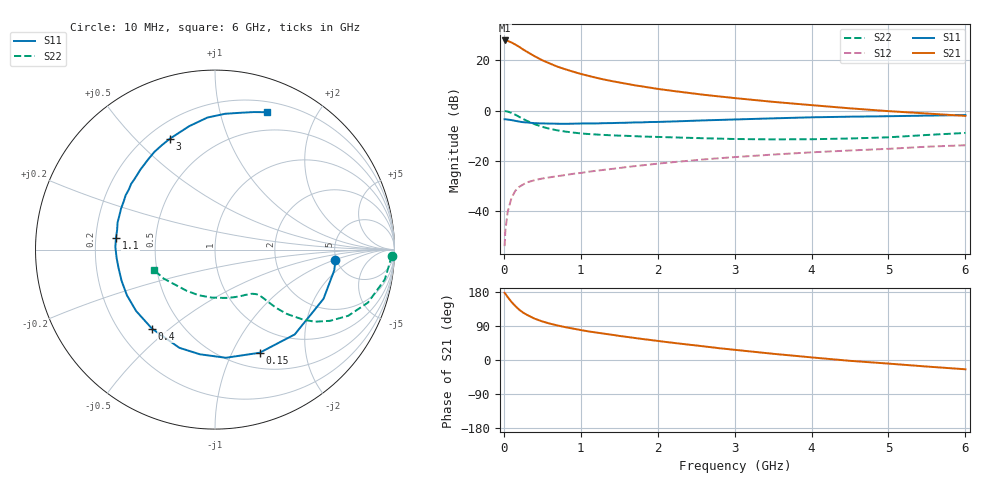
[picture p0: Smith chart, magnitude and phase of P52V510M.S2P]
! SIEMENS Small Signal Semiconductors
! BFP183
! Si NPN RF Bipolar Junction Transistor in SOT143
! VCE = 2.5 V  IC = 10 mA
! Common Emitter S-Parameters:  March  1996
# GHz  S  MA  R  50
!  f  S11  S21  S12  S22
! GHz  MAG  ANG  MAG  ANG  MAG  ANG  MAG  ANG
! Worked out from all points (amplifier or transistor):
!   36 points, 10 MHz to 6 GHz, reference 50 ohm
!   highest |S21| = 28.0 dB at 10 MHz (marker M1)
!   |S21| within 3 dB of that: start of sweep to 222.3 MHz
!   unconditionally stable (mu >= 1): 1.144 GHz to 5.571 GHz
!   at 250 MHz: K = 0.33, MSG = 26.9 dB, |S12| = -29.4 dB
!   at 1.4 GHz: K = 1.09, MAG = 15.7 dB, |S12| = -23.2 dB
!   at 6 GHz: K = 0.95, MSG = 5.8 dB, |S12| = -13.8 dB
!   lowest NFmin = 1.30 dB at 450 MHz
!   S11 on the Smith chart (normalised r, x): 10 MHz: 4.91, -1.01; 150 MHz: 0.68, -1.28; 400 MHz: 0.34, -0.44; 1.1 GHz: 0.29, +0.05; 3 GHz: 0.29, +0.63; 6 GHz: 0.30, +1.40
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0.01  0.6737 -4.8  25.01 177.2  0.002 82.8  0.9842 -2.0
0.02  0.6744 -9.8  24.98 174.7  0.0041 85.6  0.9774 -4.1
0.05  0.6639 -24.4  24.54 166.0  0.0097 79.9  0.9605 -10.0
0.1  0.6486 -46.8  22.76 153.2  0.0184 68.8  0.9021 -19.1
0.15  0.6262 -66.6  20.7 142.1  0.0254 60.9  0.829 -26.4
0.2  0.6057 -84.3  18.67 132.7  0.0303 55.9  0.7533 -31.8
0.25  0.5893 -98.2  16.57 125.1  0.0338 51.0  0.685 -35.9
0.3  0.5821 -109.9  14.9 119.3  0.0373 47.8  0.6261 -38.5
0.4  0.5632 -128.5  12.14 109.1  0.0412 44.1  0.5382 -41.8
0.5  0.557 -142.1  10.07 101.8  0.0445 41.4  0.476 -43.5
0.6  0.5528 -152.6  8.676 95.9  0.0471 41.2  0.4337 -44.2
0.7  0.5488 -161.5  7.485 91.0  0.0497 41.2  0.4038 -44.7
0.9  0.55 -175.0  5.986 82.9  0.0552 41.4  0.3661 -45.5
1.1  0.5556 173.5  4.937 75.5  0.0607 42.5  0.3423 -46.8
1.5  0.5712 156.4  3.641 63.6  0.0721 43.5  0.318 -50.9
1.8  0.5851 145.2  3.033 55.4  0.0815 43.4  0.3057 -55.3
2.2  0.6096 132.9  2.469 45.3  0.0942 42.3  0.2937 -62.5
3  0.6671 112.1  1.781 26.9  0.1188 38.3  0.2725 -80.8
3.5  0.7026 101.8  1.498 16.4  0.1335 35.2  0.268 -94.2
4.5  0.7587 85.8  1.113 -2.2  0.161 27.8  0.2787 -124.7
5.5  0.7964 74.2  0.878 -17.3  0.1915 20.9  0.3279 -150.4
6  0.8178 69.4  0.786 -24.5  0.2046 16.5  0.3598 -161.9
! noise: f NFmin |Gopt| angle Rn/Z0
0.45  1.3  0.15  45  0.18
0.9  1.4  0.2  125  0.19
1.8  2.1  0.34  -170  0.14
